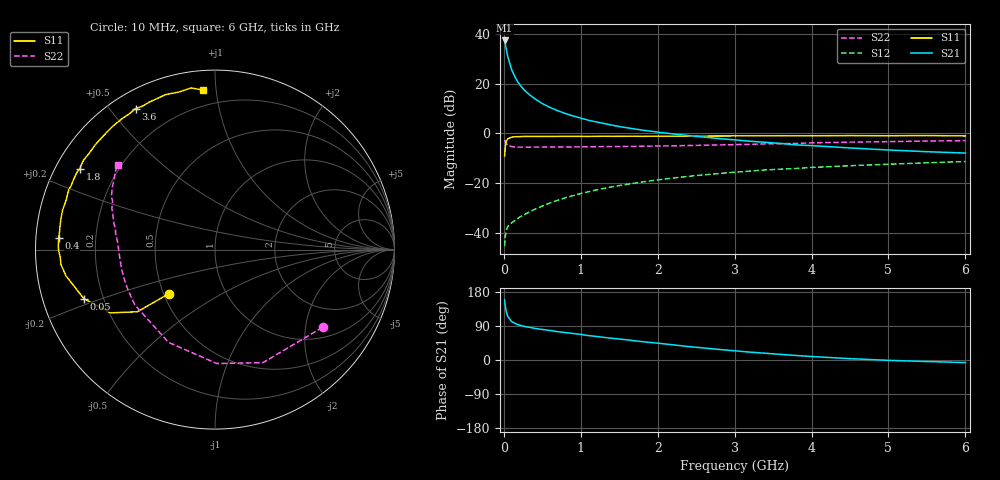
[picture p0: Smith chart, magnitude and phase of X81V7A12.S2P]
! SIEMENS Small Signal Semiconductors
! BFP136W
! Si NPN RF Bipolar Junction Transistor in SOT343
! VCE = 1.75 V  IC = 120 mA
! Common Emitter S-Parameters:  September  1994
# GHz  S  MA  R  50
!  f  S11  S21  S12  S22
! GHz  MAG  ANG  MAG  ANG  MAG  ANG  MAG  ANG
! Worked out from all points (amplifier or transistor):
!   40 points, 10 MHz to 6 GHz, reference 50 ohm
!   highest |S21| = 37.4 dB at 10 MHz (marker M1)
!   |S21| within 3 dB of that: start of sweep to 28.64 MHz
!   unconditionally stable (mu >= 1): 432.2 MHz to 3.111 GHz; 5.9902 GHz to end of sweep
!   at 200 MHz: K = 0.76, MSG = 26.8 dB, |S12| = -33.8 dB
!   at 1.5 GHz: K = 1.12, MAG = 9.8 dB, |S12| = -21.0 dB
!   at 6 GHz: K = 1.00, MAG = 1.5 dB, |S12| = -11.3 dB
!   S11 on the Smith chart (normalised r, x): 10 MHz: 0.54, -0.30; 50 MHz: 0.13, -0.18; 400 MHz: 0.07, +0.04; 1.8 GHz: 0.07, +0.28; 3.6 GHz: 0.07, +0.58; 6 GHz: 0.11, +0.92
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0.01  0.3535 -136.2  74.53 158.3  0.0054 65.7  0.7398 -35.8
0.02  0.5539 -141.3  62.34 140.9  0.0086 53.5  0.6842 -67.0
0.03  0.6807 -148.8  51.4 129.0  0.0111 46.8  0.6348 -89.1
0.05  0.7802 -159.5  35.81 115.4  0.0134 37.8  0.5782 -116.6
0.1  0.843 -170.0  19.48 101.9  0.0159 36.4  0.5428 -145.4
0.15  0.8623 -174.5  13.19 95.9  0.018 41.8  0.5337 -156.7
0.2  0.8633 -177.2  9.889 92.2  0.0205 45.1  0.5315 -162.6
0.25  0.8714 -179.7  7.975 89.4  0.0226 48.3  0.5316 -166.5
0.3  0.8732 178.9  6.657 87.4  0.0248 51.1  0.5307 -169.1
0.4  0.8732 175.7  5.017 83.6  0.0298 55.1  0.5315 -172.6
0.5  0.8718 173.1  4.001 80.5  0.0346 58.1  0.5326 -175.0
0.6  0.8735 171.3  3.338 77.9  0.04 60.2  0.5334 -176.7
0.7  0.8748 168.9  2.878 74.8  0.0453 61.7  0.5349 -177.8
0.9  0.8767 165.5  2.254 69.9  0.0562 62.8  0.537 179.7
1.1  0.874 161.3  1.849 64.4  0.0673 62.8  0.5402 178.1
1.8  0.8767 149.0  1.17 48.4  0.1059 59.2  0.5524 172.3
2.2  0.8829 142.4  0.979 40.0  0.1269 55.7  0.5642 169.2
3.2  0.8947 125.5  0.699 20.8  0.1751 45.7  0.6054 160.1
3.6  0.9017 119.4  0.63 14.9  0.1917 41.7  0.624 156.6
4.5  0.9063 107.7  0.512 3.6  0.2245 33.0  0.6701 148.6
5.5  0.9106 98.4  0.43 -4.0  0.2572 24.9  0.7049 142.0
6  0.8909 94.2  0.404 -6.8  0.2731 20.6  0.7182 139.1
